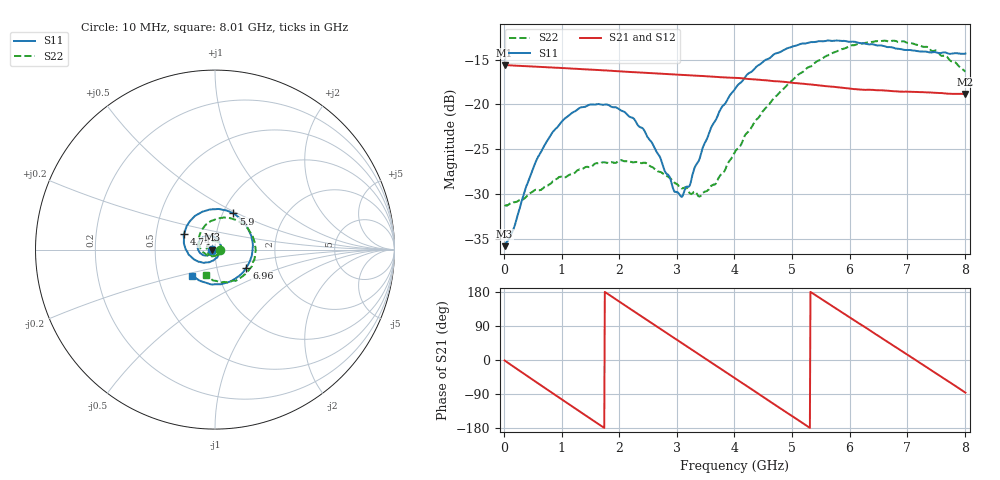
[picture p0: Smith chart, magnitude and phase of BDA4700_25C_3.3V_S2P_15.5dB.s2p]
!Agilent Technologies,E5071B,MY42404982,A.09.10
!Date: Mon Oct 20 18:09:32 2025
!Data & Calibration Information:
!Freq	S11:SOLT2(ON)	S21:SOLT2(ON)	S12:SOLT2(ON)	S22:SOLT2(ON)
# Hz S RI R 50
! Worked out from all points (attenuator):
!   801 points, 10 MHz to 8.01 GHz, reference 50 ohm
!   highest |S21| = -15.59 dB at 10 MHz (marker M1); lowest = -18.8 dB at 8.01 GHz (marker M2)
!   lowest |S11| = -35.8 dB at 10 MHz (marker M3), VSWR 1.03, Z = 48.4 - j0.109 ohm
!   |S11| at or under -10 dB: start of sweep to end of sweep
!   |S22| runs from -31.3 to -12.9 dB; largest |S21 - S12| = 0.0019
!   S11 on the Smith chart (normalised r, x): 10 MHz: 0.97, -0.00; 4.74 GHz: 0.70, +0.13; 5.9 GHz: 1.12, +0.48; 6.96 GHz: 1.39, -0.29; 8.01 GHz: 0.75, -0.23
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1e7  -0.0161 -0.00113  0.166 -0.0036  0.1659 -0.00377  0.0274 -0.000995
1.5e8  -0.0172 -0.00956  0.1583 -0.0453  0.1582 -0.0453  0.0272 -0.00773
4e8  -0.0259 -0.0246  0.1214 -0.1091  0.1214 -0.1091  0.021 -0.0227
7e8  -0.0484 -0.0335  0.0474 -0.1543  0.0476 -0.1542  0.00433 -0.0343
1.03e9  -0.0786 -0.0231  -0.0459 -0.1527  -0.0459 -0.1526  -0.0202 -0.0336
1.35e9  -0.0962 0.00623  -0.1196 -0.102  -0.1196 -0.1023  -0.041 -0.0147
2.08e9  -0.0504 0.076  -0.1266 0.0848  -0.1267 0.0848  -0.0245 0.0415
2.42e9  -0.00572 0.0724  -0.0557 0.1394  -0.0558 0.1393  0.00567 0.0468
2.68e9  0.0212 0.048  0.0113 0.1482  0.011 0.148  0.0243 0.0345
2.96e9  0.0313 0.00884  0.0787 0.1237  0.0785 0.1235  0.034 0.0135
3.09e9  0.0288 -0.0102  0.1046 0.102  0.1036 0.1025  0.0339 0.00114
3.41e9  0.000728 -0.0516  0.1408 0.0309  0.1409 0.0309  0.019 -0.0242
3.75e9  -0.0568 -0.0732  0.1317 -0.0526  0.1319 -0.0526  -0.0138 -0.0376
4.01e9  -0.1058 -0.0605  0.0939 -0.1045  0.094 -0.1043  -0.0446 -0.0307
4.74e9  -0.1725 0.0869  -0.071 -0.1142  -0.0704 -0.1146  -0.0888 0.0688
5.35e9  -0.0638 0.2132  -0.1286 0.00704  -0.1287 0.00634  -0.00757 0.1644
5.9e9  0.1025 0.2013  -0.0657 0.1048  -0.066 0.1043  0.1292 0.1586
6.35e9  0.1948 0.0934  0.0242 0.1182  0.0241 0.1175  0.2118 0.068
6.68e9  0.2082 -0.0144  0.083 0.0852  0.0833 0.0851  0.2236 -0.0244
6.96e9  0.1748 -0.0999  0.1117 0.0373  0.1117 0.0365  0.1999 -0.0995
7.48e9  0.0344 -0.1925  0.097 -0.0638  0.0971 -0.064  0.0789 -0.1833
8.01e9  -0.1255 -0.1456  0.00766 -0.1139  0.00796 -0.1139  -0.051 -0.1434
